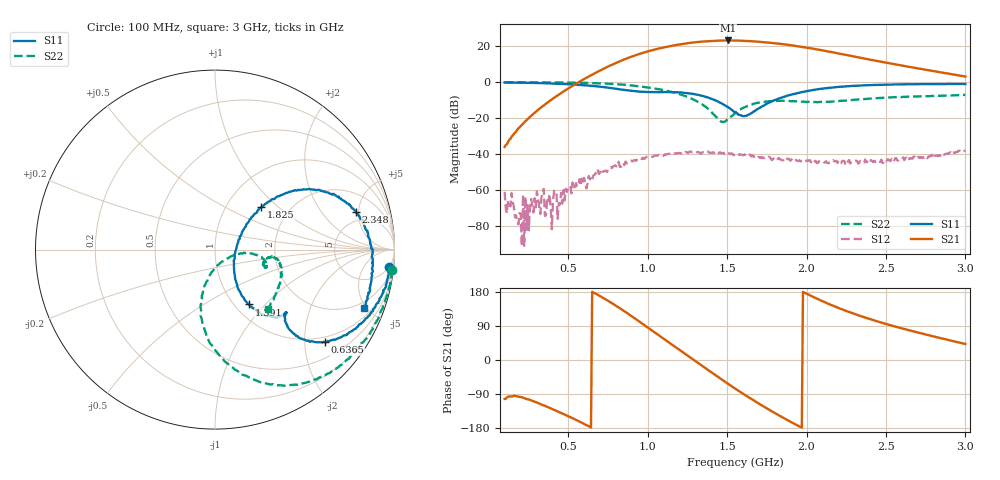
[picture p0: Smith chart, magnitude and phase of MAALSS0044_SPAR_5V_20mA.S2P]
!Part No: MAALSS0044
!Bias: Vdd=5V, Idd=20mA (R1=39ohms)
!2-port de-embedded S-parameters
!Date: Wed Sep 14 15:55:45 20111
!Temp: +25c
!REF Task A17L_2309
!Fixture: 25050XX Rev00
!Test System: Agilent Technologies,E5071C,MY46106711,A.09.61
!Data & Calibration Information:
!Freq	S11:SOLT2(ON)	S21:SOLT2(ON)	S12:SOLT2(ON)	S22:SOLT2(ON)
!PortZ  Port1:50+j0  Port2:50+j0
# Hz S dB R 50
!Freq(Hz)	S11(dB) 	S11(Angle)	S21(dB) 	S21(Angle)	S12(dB) 	S12(Angle)	S22(dB) 	S22(Angle)
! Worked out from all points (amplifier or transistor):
!   401 points, 100 MHz to 3 GHz, reference 50 ohm
!   highest |S21| = 23.3 dB at 1.506 GHz (marker M1)
!   |S21| within 3 dB of that: 1.152 GHz to 1.929 GHz (776.9 MHz wide, 50.4 % of centre)
!   unconditionally stable (mu >= 1): start of sweep to end of sweep
!   at 578.5 MHz: K = 7.57, MAG = 17.4 dB, |S12| = -57.7 dB
!   at 1.55 GHz: K = 3.34, MAG = 23.4 dB, |S12| = -39.9 dB
!   at 3 GHz: K = 4.48, MAG = 11.2 dB, |S12| = -38.2 dB
!   S11 on the Smith chart (normalised r, x): 100 MHz: 4, -19; 636.5 MHz: 0.87, -2.48; 1.391 GHz: 1.16, -0.81; 1.825 GHz: 1.45, +0.78; 2.348 GHz: 3.74, +4.66; 3 GHz: 1.53, -4.81
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1e8  -0.21 -5.8  -36.11 -102.8  -61.11 13.2  -0.04 -6.6
5.8575e8  -1.57 -37.0  0.99 -165.5  -53.78 169.2  -0.36 -39.6
6.365e8  -1.94 -40.1  3.50 -176.7  -54.18 176.9  -0.45 -43.7
7.5975e8  -3.16 -45.7  9.07 154.1  -47.82 141.5  -0.88 -54.4
8.83e8  -4.66 -46.5  13.71 120.4  -44.48 132.4  -1.68 -66.3
9.7e8  -5.38 -43.6  16.36 95.0  -42.04 110.0  -2.57 -74.6
1.0715e9  -5.58 -41.4  18.77 65.0  -40.38 94.7  -3.97 -84.2
1.16575e9  -5.57 -43.6  20.50 37.0  -39.99 77.7  -5.72 -93.4
1.26e9  -6.19 -49.7  21.83 9.0  -39.02 59.2  -8.46 -102.3
1.32525e9  -7.21 -54.8  22.48 -10.3  -39.13 38.8  -11.44 -106.0
1.3905e9  -8.89 -58.4  22.92 -29.3  -39.39 32.3  -15.62 -103.3
1.5065e9  -13.97 -55.8  23.26 -62.8  -39.25 5.6  -20.82 -27.3
1.55e9  -16.62 -44.0  23.23 -75.0  -39.92 -7.5  -17.33 -10.1
1.666e9  -16.38 24.1  22.75 -106.4  -41.47 -37.8  -12.08 -8.7
1.74575e9  -12.22 39.5  22.20 -126.5  -41.82 -56.0  -10.72 -13.4
1.8255e9  -9.10 42.5  21.47 -145.9  -42.29 -82.9  -10.39 -17.6
1.91975e9  -6.63 39.7  20.38 -167.5  -42.94 -99.8  -10.57 -19.5
2.03575e9  -4.47 34.2  18.76 168.0  -43.83 -127.1  -10.94 -16.2
2.16625e9  -2.96 26.0  16.64 143.3  -43.39 -155.8  -10.79 -10.0
2.3475e9  -1.80 15.0  13.51 114.9  -44.31 -177.2  -9.46 -8.1
2.5215e9  -1.35 5.2  10.52 92.4  -43.77 -167.1  -8.57 -14.0
3e9  -1.01 -21.5  3.17 42.4  -38.19 -169.7  -7.05 -48.3
